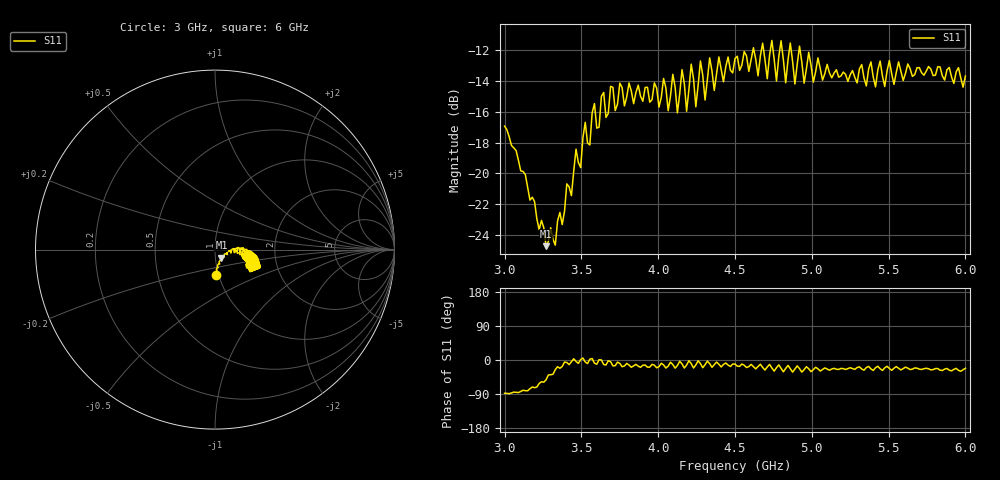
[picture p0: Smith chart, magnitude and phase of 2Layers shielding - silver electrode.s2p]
!  03/07/2025  15:32:00
! Ref Plane: 0.000 mm
# MHZ S MA R  50
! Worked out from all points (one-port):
!   201 points, 3 GHz to 6 GHz, reference 50 ohm
!   lowest |S11| = -24.7 dB at 3.27 GHz (marker M1), VSWR 1.12, Z = 53.5 - j4.91 ohm
!   |S11| at or under -10 dB: start of sweep to end of sweep
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3000  0.1424 -87.9
3270  0.05803 -52.1
3375  0.06821 -17.2
3525  0.1465 -5.3
3555  0.1237 2.2
3585  0.1686 -8.4
3615  0.1413 0.7
3630  0.1779 0.2
3750  0.1964 -9.0
4005  0.1642 -17.6
4035  0.2034 -13.1
4065  0.1599 -16.1
4095  0.2098 -11.9
4125  0.1573 -14.6
4155  0.2173 -10.2
4185  0.1592 -13.3
4215  0.2264 -9.6
4245  0.1646 -13.1
4275  0.2319 -9.5
4305  0.1732 -12.5
4335  0.2373 -9.6
4365  0.186 -12.3
4395  0.2389 -11.2
4500  0.2361 -10.8
4875  0.2312 -32.1
5250  0.2091 -20.3
5625  0.2267 -21.5
6000  0.2071 -22.1
